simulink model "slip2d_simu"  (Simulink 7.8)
settings: Solver=ode45  StartTime=0.0  StopTime=10.0  FixedStep=1e-4  MaxStep=0.01  RelTol=1e-3
undefined symbols (not defined in the file or in its folder): MP

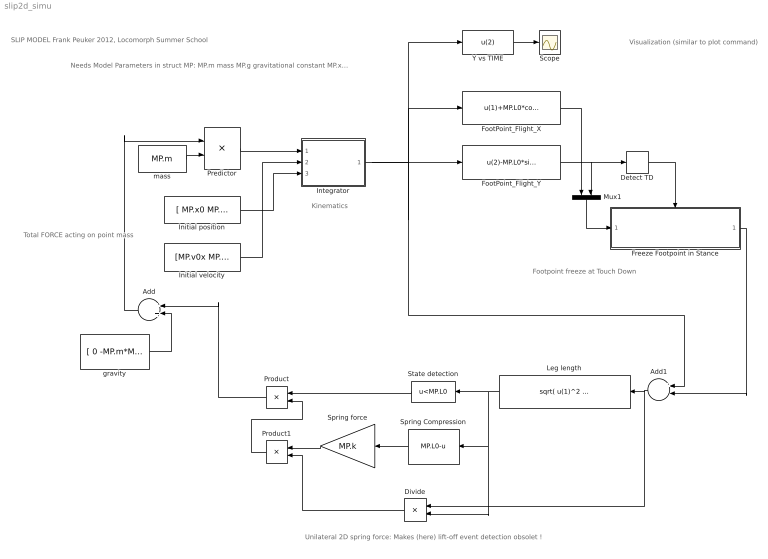
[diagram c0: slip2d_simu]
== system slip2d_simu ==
  note: Total FORCE acting on point mass
  note: Kinematics
  note: Footpoint freeze at Touch Down
  note: Unilateral 2D spring force: Makes (here) lift-off event detection obsolet !
  note: Visualization (similar to plot command)
  note: Needs Model Parameters in struct MP: MP.m mass MP.g gravitational constant MP.x0 MP.y0 initial position MP.v0x MP.v0y initial speed MP.L0 rest leg length (e.g. in standing) MP.k stiffness of spring MP.alpha Angle of attack
  note: SLIP MODEL Frank Peuker 2012, Locomorph Summer School
  Add : Sum
  Add1 : Sum  Inputs=+-
  Detect TD : HitCross  HitCrossingDirection=falling
  Divide : Product  Inputs=*/
  FootPoint_Flight_X : Fcn  Expr=u(1)+MP.L0*cos(MP.alpha)
  FootPoint_Flight_Y : Fcn  Expr=u(2)-MP.L0*sin(MP.alpha)
  Freeze Footpoint in Stance : Subsystem  TreatAsAtomicUnit=on
  Initial position : Constant  Value=[ MP.x0 MP.y0]
  Initial velocity : Constant  Value=[MP.v0x MP.v0y]
  Integrator : Subsystem
  Leg length : Fcn  Expr=sqrt( u(1)^2 + u(2)^2 )
  Mux1 : Mux  Inputs=2
  Predictor : Product  Inputs=*/
  Product : Product
  Product1 : Product
  Scope : Scope
  Spring Compression : Fcn  Expr=MP.L0-u
  Spring force : Gain  Gain=MP.k
  State detection : Fcn  Expr=u<MP.L0
  Y vs TIME : Fcn  Expr=u(2)
  gravity : Constant  Value=[ 0 -MP.m*MP.g]
  mass : Constant  Value=MP.m
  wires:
  Initial velocity/1 -> Integrator/2(v_init)
  Initial position/1 -> Integrator/3(L_init)
  Predictor/1 -> Integrator/1(a)
  mass/1 -> Predictor/2
  Integrator/1(r) -> FootPoint_Flight_X/1, FootPoint_Flight_Y/1, Add1/1, Y vs TIME/1
  Add/1 -> Predictor/1
  gravity/1 -> Add/2
  State detection/1 -> Product/1
  Product/1 -> Add/1
  Detect TD/1 -> Freeze Footpoint in Stance/Trigger
  Freeze Footpoint in Stance/1(FootPoint_Stance) -> Add1/2
  Mux1/1 -> Freeze Footpoint in Stance/1(FootPoint_Flight)
  FootPoint_Flight_X/1 -> Mux1/1
  Leg length/1 -> State detection/1, Divide/2, Spring Compression/1
  Spring force/1 -> Product1/1
  Divide/1 -> Product1/2
  Product1/1 -> Product/2
  Y vs TIME/1 -> Scope/1
  Spring Compression/1 -> Spring force/1
  Add1/1 -> Leg length/1, Divide/1
  FootPoint_Flight_Y/1 -> Detect TD/1, Mux1/2

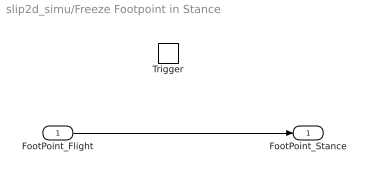
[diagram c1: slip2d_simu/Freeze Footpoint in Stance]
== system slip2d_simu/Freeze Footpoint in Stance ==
  FootPoint_Flight : Inport
  Trigger : TriggerPort
  FootPoint_Stance : Outport  InitialOutput=[-100 0]
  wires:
  FootPoint_Flight/1 -> FootPoint_Stance/1

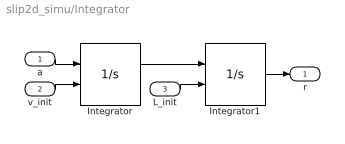
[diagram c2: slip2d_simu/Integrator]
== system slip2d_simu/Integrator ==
  a : Inport
  v_init : Inport  Port=2
  L_init : Inport  Port=3
  Integrator : Integrator  InitialConditionSource=external
  Integrator1 : Integrator  InitialConditionSource=external
  r : Outport
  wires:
  Integrator/1 -> Integrator1/1
  a/1 -> Integrator/1
  Integrator1/1 -> r/1
  v_init/1 -> Integrator/2
  L_init/1 -> Integrator1/2
